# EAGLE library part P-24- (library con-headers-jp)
HEADER PLUG PINS
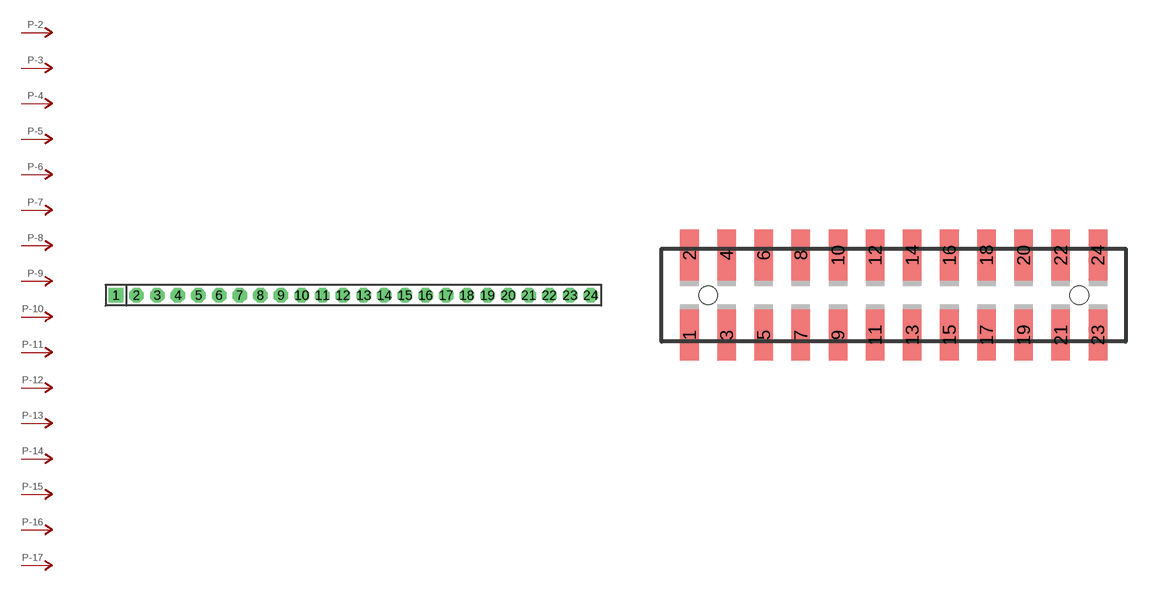
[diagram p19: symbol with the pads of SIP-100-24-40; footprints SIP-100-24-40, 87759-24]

Designator prefix P; gates -2=P-N -3=P-N -4=P-N -5=P-N -6=P-N -7=P-N -8=P-N -9=P-N -10=P-N -11=P-N -12=P-N -13=P-N -14=P-N -15=P-N -16=P-N -17=P-N -18=P-N -19=P-N -20=P-N -21=P-N -22=P-N -23=P-N -24=P-N -1=P-NV

## P-24-SIP-100-40  [SIP-100-24-40]
1  -1:P  pas
2  -2:P  pas
3  -3:P  pas
4  -4:P  pas
5  -5:P  pas
6  -6:P  pas
7  -7:P  pas
8  -8:P  pas
9  -9:P  pas
10  -10:P  pas
11  -11:P  pas
12  -12:P  pas
13  -13:P  pas
14  -14:P  pas
15  -15:P  pas
16  -16:P  pas
17  -17:P  pas
18  -18:P  pas
19  -19:P  pas
20  -20:P  pas
21  -21:P  pas
22  -22:P  pas
23  -23:P  pas
24  -24:P  pas

## P-24-87759  [87759-24]
Pads as for SIP-100-24-40

## P-24-100-2X12  [DIL-100-2X12]
Pads as for SIP-100-24-40

## P-24-100-2X12_M  [DIL-100-2X12_M]
Pads as for SIP-100-24-40

## P-24-2MM-2X12  [DIL-2MM-2X12]
Pads as for SIP-100-24-40

## P-24-2MM-2X12_M  [DIL-2MM-2X12_M]
Pads as for SIP-100-24-40

## P-24-SIP-100-32  [SIP-100-24-32]
Pads as for SIP-100-24-40

## P-24-SIP-100-40Y  [SIP-100-24-40Y]
Pads as for SIP-100-24-40

## P-24-SIP-100-32Y  [SIP-100-24-32Y]
Pads as for SIP-100-24-40

## P-24-87759_M  [87759-24_M]
Pads as for SIP-100-24-40

## Footprint SIP-100-24-40 (pad centres in mm)
SIP Header - 0.1", 40 mil drill
drill 1.016 pad 1.778 square: 1 -29.21,0
drill 1.016 pad 1.778 octagon: 2 -26.67,0; 3 -24.13,0; 4 -21.59,0; 5 -19.05,0; 6 -16.51,0; 7 -13.97,0; 8 -11.43,0; 9 -8.89,0; 10 -6.35,0; 11 -3.81,0; 12 -1.27,0; 13 1.27,0; 14 3.81,0; 15 6.35,0; 16 8.89,0; 17 11.43,0; 18 13.97,0; 19 16.51,0; 20 19.05,0; 21 21.59,0; 22 24.13,0; 23 26.67,0; 24 29.21,0

## Footprint 87759-24 (pad centres in mm)
Molex PCB Pin Headers 2.00mm (.079") Pitch Milli-Grid Header, Vertical SMD
smd 1 x 2.75: 1 -11,-2.15; 2 -11,2.15; 3 -9,-2.15; 4 -9,2.15; 5 -7,-2.15; 6 -7,2.15; 7 -5,-2.15; 8 -5,2.15; 9 -3,-2.15; 10 -3,2.15; 11 -1,-2.15; 12 -1,2.15; 13 1,-2.15; 14 1,2.15; 15 3,-2.15; 16 3,2.15; 17 5,-2.15; 18 5,2.15; 19 7,-2.15; 20 7,2.15; 21 9,-2.15; 22 9,2.15; 23 11,-2.15; 24 11,2.15
hole 1 at -10,0
hole 1 at 10,0

## Footprint DIL-100-2X12 (pad centres in mm)
PIN HEADER - 0.1"
drill 1.016 square: 1 -13.97,-1.27
drill 1.016 octagon: 2 -13.97,1.27; 3 -11.43,-1.27; 4 -11.43,1.27; 5 -8.89,-1.27; 6 -8.89,1.27; 7 -6.35,-1.27; 8 -6.35,1.27; 9 -3.81,-1.27; 10 -3.81,1.27; 11 -1.27,-1.27; 12 -1.27,1.27; 13 1.27,-1.27; 14 1.27,1.27; 15 3.81,-1.27; 16 3.81,1.27; 17 6.35,-1.27; 18 6.35,1.27; 19 8.89,-1.27; 20 8.89,1.27; 21 11.43,-1.27; 22 11.43,1.27; 23 13.97,-1.27; 24 13.97,1.27

## Footprint DIL-100-2X12_M (pad centres in mm)
PIN HEADER - MIRRORED 0.1"
drill 1.016 square: 1 -13.97,1.27
drill 1.016 octagon: 2 -13.97,-1.27; 3 -11.43,1.27; 4 -11.43,-1.27; 5 -8.89,1.27; 6 -8.89,-1.27; 7 -6.35,1.27; 8 -6.35,-1.27; 9 -3.81,1.27; 10 -3.81,-1.27; 11 -1.27,1.27; 12 -1.27,-1.27; 13 1.27,1.27; 14 1.27,-1.27; 15 3.81,1.27; 16 3.81,-1.27; 17 6.35,1.27; 18 6.35,-1.27; 19 8.89,1.27; 20 8.89,-1.27; 21 11.43,1.27; 22 11.43,-1.27; 23 13.97,1.27; 24 13.97,-1.27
